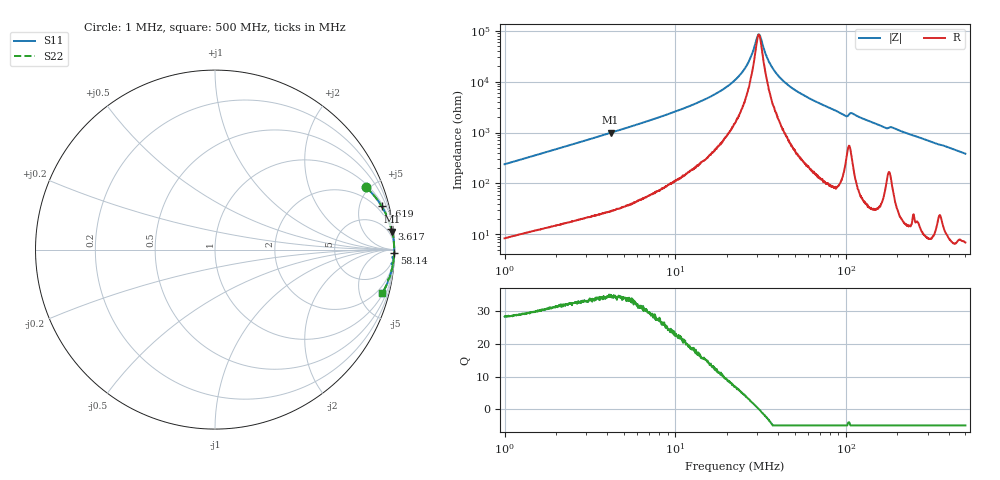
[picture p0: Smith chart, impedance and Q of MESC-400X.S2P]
!s-Parameter Generated by FASTRON Sdn. Bhd.
!FASTRON P/N : MESC-400X
!Keysight Technologies,E4991B,MY54100416,A.01.15
!Date: Mon Mar 16 11:14:08 2026
!Version  : Rev00 Mon Mar 16 11:14:08 2026
!Data & Calibration Information:
!PortZ  Port1:50+j0  Port2:50+j0
!When reading, reference impedance value at option line is always used.
!Remarks : This data is being provided solely for informational purposes.
!Freq	S11	S21	S12	S22
# Hz S dB R 50
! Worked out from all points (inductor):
!   1601 points, 1 MHz to 500 MHz, reference 50 ohm
!   read as one part in series: L = 37.6 uH near 1.032 MHz
!   highest Q = 34.7 at 4.176 MHz (marker M1), where L = 37.6 uH
!   self-resonance near 30.75 MHz
!   S11 on the Smith chart (normalised r, x): 1 MHz: 1.17, +4.76; 1.619 MHz: 1.25, +7.63; 3.617 MHz: 2, +17; 58.14 MHz: open; 500 MHz: 1.14, -7.68
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1000000  -0.81 22.5  -8.35 -65.5  -8.35 -65.5  -0.81 22.5
1618714  -0.36 14.6  -11.99 -73.5  -11.99 -73.5  -0.36 14.6
2820919  -0.14 8.6  -16.55 -79.7  -16.55 -79.7  -0.14 8.6
3617008  -0.09 6.7  -18.68 -81.6  -18.68 -81.6  -0.09 6.7
4176025  -0.07 5.8  -19.95 -82.6  -19.95 -82.6  -0.07 5.8
7957584  -0.03 2.9  -25.91 -85.0  -25.91 -85.0  -0.03 2.9
1.534122e7  -0.01 1.2  -33.42 -84.9  -33.42 -84.9  -0.01 1.2
2.236068e7  -0.01 0.5  -40.60 -81.3  -40.60 -81.3  -0.01 0.5
2.622081e7  -0.01 0.3  -46.45 -74.2  -46.45 -74.2  -0.01 0.3
2.801062e7  -0.01 0.2  -50.41 -65.3  -50.41 -65.3  -0.01 0.2
3.003904e7  -0.01 0.0  -57.01 -31.5  -57.01 -31.5  -0.01 0.0
3.09871e7  -0.01 -0.0  -58.31 7.1  -58.31 7.1  -0.01 -0.0
3.171773e7  -0.01 -0.0  -57.04 35.3  -57.04 35.3  -0.01 -0.0
3.508814e7  -0.01 -0.2  -48.24 72.0  -48.24 72.0  -0.01 -0.2
3.896776e7  -0.01 -0.4  -43.28 80.0  -43.28 80.0  -0.01 -0.4
4.641026e7  -0.01 -0.7  -38.32 84.9  -38.32 84.9  -0.01 -0.7
5.813687e7  -0.01 -1.1  -34.13 86.2  -34.13 86.2  -0.01 -1.1
6.307767e7  -0.01 -1.3  -32.90 86.4  -32.90 86.4  -0.01 -1.3
9.859709e7  -0.05 -2.6  -26.67 81.6  -26.67 81.6  -0.05 -2.6
1.086514e8  -0.05 -2.4  -27.56 81.0  -27.56 81.0  -0.05 -2.4
1.77937e8  -0.12 -4.5  -21.97 77.7  -21.97 77.7  -0.12 -4.5
5e8  -0.32 -14.5  -12.01 74.4  -12.01 74.4  -0.32 -14.5
